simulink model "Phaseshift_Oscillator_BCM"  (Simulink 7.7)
settings: Solver=ode113  StartTime=0.0  StopTime=100  FixedStep=1e-4  RelTol=3e-14
libraries: fl_lib x12, nesl_utility x3, Memristor_lib x1

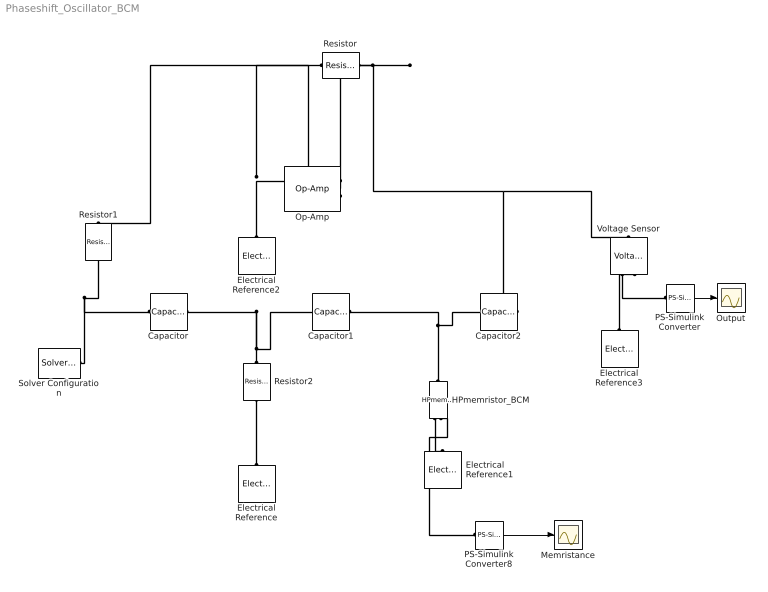
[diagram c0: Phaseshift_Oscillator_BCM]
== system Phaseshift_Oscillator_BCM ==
  Capacitor : fl_lib/Electrical/Electrical Elements/Capacitor  SystemSampleTime=-1  c=1e-6 F  v0=.1 V  r=1e-6 Ohm  g=0 1/Ohm  i_Log=off  v_Log=off  vc_Log=off  LocalVarNames=|i|v|vc  LocalVarDescs=|i|v|Internal variable for voltage across capacitor term  LocalVarLogging=[0 0 0]
  Capacitor1 : fl_lib/Electrical/Electrical Elements/Capacitor  SystemSampleTime=-1  c=1e-6 F  v0=0 V  r=1e-6 Ohm  g=0 1/Ohm  i_Log=off  v_Log=off  vc_Log=off  LocalVarNames=|i|v|vc  LocalVarDescs=|i|v|Internal variable for voltage across capacitor term  LocalVarLogging=[0 0 0]
  Capacitor2 : fl_lib/Electrical/Electrical Elements/Capacitor  SystemSampleTime=-1  c=1e-6 F  v0=0 V  r=1e-6 Ohm  g=0 1/Ohm  i_Log=off  v_Log=off  vc_Log=off  LocalVarNames=|i|v|vc  LocalVarDescs=|i|v|Internal variable for voltage across capacitor term  LocalVarLogging=[0 0 0]
  Electrical Reference{,1..3} (4 alike) : fl_lib/Electrical/Electrical Elements/Electrical Reference  SystemSampleTime=-1  i_Log=off  LocalVarNames=|i  LocalVarDescs=|i  LocalVarLogging=0
  HPmemristor_BCM : Memristor_lib/HPmemristor_BCM  SystemSampleTime=-1  G_off=6.25e-5 1/Ohm  G_on=2e-3 1/Ohm  N=1 1/Ohm  u_v=1e-10 m^2/s/V  D=1e-8 m  x0=.5 Ohm  t0=1 s  i0=1 A  VT1=0 V  VT0=0 V  i_Log=off  v_Log=off  x_Log=off  F_Log=off  W_Log=off  LocalVarNames=|i|v|x|F|W  LocalVarDescs=|i|v|x|F|W  LocalVarLogging=[0 0 0 0 0]
  Memristance : Scope
  Op-Amp : fl_lib/Electrical/Electrical Elements/Op-Amp  SystemSampleTime=-1  i1_Log=off  v1_Log=off  outI_Log=off  LocalVarNames=|i1|v1|outI  LocalVarDescs=|i1|v1|outI  LocalVarLogging=[0 0 0]
  Output : Scope
  PS-Simulink Converter : nesl_utility/PS-Simulink Converter  SystemSampleTime=-1  PhysicalDomain=network_engine_domain  LeftPortType=input  RightPortType=output  SubClassName=ps_output  Unit=1  AffineConversion=off
  PS-Simulink Converter8 : nesl_utility/PS-Simulink Converter  SystemSampleTime=-1  PhysicalDomain=network_engine_domain  LeftPortType=input  RightPortType=output  SubClassName=ps_output  Unit=1  AffineConversion=off
  Resistor : fl_lib/Electrical/Electrical Elements/Resistor  SystemSampleTime=-1  R=188.5 kOhm  i_Log=off  v_Log=off  LocalVarNames=|i|v  LocalVarDescs=|i|v  LocalVarLogging=[0 0]
  Resistor1 : fl_lib/Electrical/Electrical Elements/Resistor  SystemSampleTime=-1  R=6.5 kOhm  i_Log=off  v_Log=off  LocalVarNames=|i|v  LocalVarDescs=|i|v  LocalVarLogging=[0 0]
  Resistor2 : fl_lib/Electrical/Electrical Elements/Resistor  SystemSampleTime=-1  R=6.5 kOhm  i_Log=off  v_Log=off  LocalVarNames=|i|v  LocalVarDescs=|i|v  LocalVarLogging=[0 0]
  Solver Configuration : nesl_utility/Solver Configuration  SystemSampleTime=-1  PhysicalDomain=network_engine_domain  LeftPortType=input  RightPortType=generic  SubClassName=solver  Accelerate=off  Profile=off  ResidualTolerance=1e-9  MaxNonlinIter=3  MaxModeIter=2  DoFixedCost=off  UseLocalSampling=off  DoDC=off  LinearAlgebra=Sparse  LocalSolverSampleTime=.001  LocalSolverChoice=NE_BACKWARD_EULER_ADVANCER  UseLocalSolver=off
  Voltage Sensor : fl_lib/Electrical/Electrical Sensors/Voltage Sensor  SystemSampleTime=-1  i1_Log=off  v1_Log=off  LocalVarNames=|i1|v1  LocalVarDescs=|i1|v1  LocalVarLogging=[0 0]
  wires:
  PS-Simulink Converter/1 -> Output/1
  PS-Simulink Converter8/1 -> Memristance/1
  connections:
  Solver Configuration/RConn1 -- Capacitor/LConn1 -- Resistor1/RConn1
  Resistor/LConn1 -- Resistor1/LConn1 -- Op-Amp/LConn2
  Resistor/RConn1 -- Op-Amp/RConn1 -- Capacitor2/RConn1 -- Voltage Sensor/LConn1
  HPmemristor_BCM/LConn1 -- Capacitor1/RConn1 -- Capacitor2/LConn1
  Resistor2/LConn1 -- Capacitor1/LConn1 -- Capacitor/RConn1
  Electrical Reference2/LConn1 -- Op-Amp/LConn1
  HPmemristor_BCM/RConn1 -- Electrical Reference1/LConn1
  Electrical Reference3/LConn1 -- Voltage Sensor/RConn2
  Voltage Sensor/RConn1 -- PS-Simulink Converter/LConn1
  Resistor2/RConn1 -- Electrical Reference/LConn1
  PS-Simulink Converter8/LConn1 -- HPmemristor_BCM/RConn2
